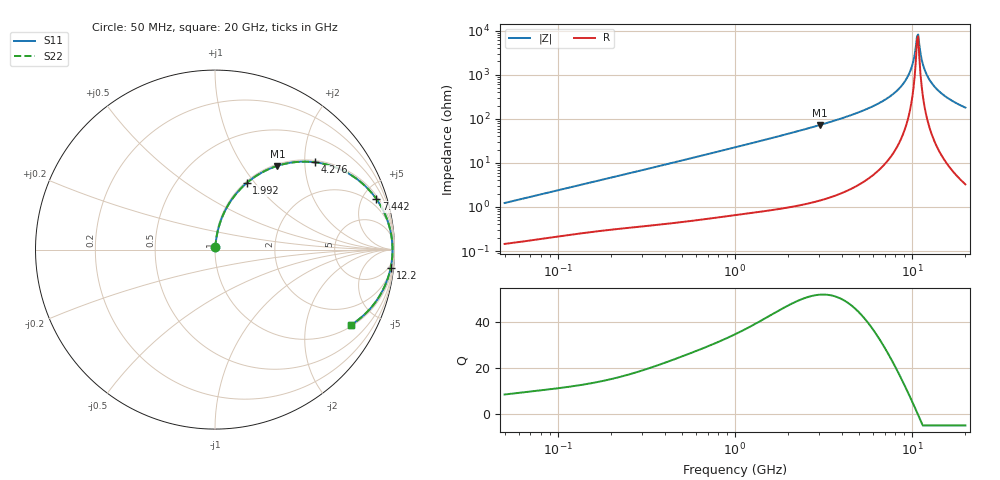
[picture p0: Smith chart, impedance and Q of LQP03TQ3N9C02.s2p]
!Murata Part Number: LQP03TQ3N9C02
!These Parameters are Measured in Series Mode Connection
!  o--[Z]--o
!Port1  Port2
!  o-------o
!Freq. Start=50[MHz] Stop=20[GHz], 401[Steps]
# Hz S RI R 50
!Freq.(Hz) S11(Real) S11(Imag) S21(Real) S21(Imag) S12(Real) S12(Imag) S22(Real) S22(Imag)
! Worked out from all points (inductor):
!   401 points, 50 MHz to 20 GHz, reference 50 ohm
!   read as one part in series: L = 3.84 nH near 51.52 MHz
!   highest Q = 51.7 at 3.03 GHz (marker M1), where L = 3.81 nH
!   self-resonance near 10.66 GHz
!   S11 on the Smith chart (normalised r, x): 50 MHz: 1.00, +0.02; 1.992 GHz: 1.02, +0.91; 4.276 GHz: 1.05, +2.24; 7.442 GHz: 1.25, +6.28; 12.2 GHz: 3, -19; 20 GHz: 1.06, -3.58
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5e7  0.00159 0.0122  0.9984 -0.0122  0.9984 -0.0122  0.00159 0.0122
1.364002e8  0.00353 0.0317  0.9965 -0.0317  0.9965 -0.0317  0.00353 0.0317
3.721004e8  0.0109 0.083  0.9891 -0.083  0.9891 -0.083  0.0109 0.083
1e9  0.0535 0.2111  0.9465 -0.2111  0.9465 -0.2111  0.0535 0.2111
1.99176e9  0.1772 0.3713  0.8228 -0.3713  0.8228 -0.3713  0.1772 0.3713
2.728004e9  0.2962 0.4469  0.7038 -0.4469  0.7038 -0.4469  0.2962 0.4469
3.029571e9  0.3477 0.4667  0.6523 -0.4667  0.6523 -0.4667  0.3477 0.4667
4.275624e9  0.5547 0.4868  0.4453 -0.4868  0.4453 -0.4868  0.5547 0.4868
5.856089e9  0.7646 0.4113  0.2354 -0.4113  0.2354 -0.4113  0.7646 0.4113
7.442007e9  0.8988 0.2824  0.1012 -0.2824  0.1012 -0.2824  0.8988 0.2824
8.516016e9  0.9514 0.1872  0.0486 -0.1872  0.0486 -0.1872  0.9514 0.1872
9.457416e9  0.9773 0.1053  0.0227 -0.1053  0.0227 -0.1053  0.9773 0.1053
1.004137e10  0.9855 0.0567  0.0145 -0.0567  0.0145 -0.0567  0.9855 0.0567
1.050288e10  0.9885 0.0197  0.0115 -0.0197  0.0115 -0.0197  0.9885 0.0197
1.066139e10  0.9889 0.00735  0.0111 -0.00735  0.0111 -0.00735  0.9889 0.00735
1.082228e10  0.989 -0.00502  0.011 0.00502  0.011 0.00502  0.989 -0.00502
1.098561e10  0.9888 -0.0174  0.0112 0.0174  0.0112 0.0174  0.9888 -0.0174
1.149051e10  0.9862 -0.0544  0.0138 0.0544  0.0138 0.0544  0.9862 -0.0544
1.220001e10  0.9784 -0.1032  0.0216 0.1032  0.0216 0.1032  0.9784 -0.1032
1.334722e10  0.9578 -0.1741  0.0422 0.1741  0.0422 0.1741  0.9578 -0.1741
1.482269e10  0.9212 -0.2512  0.0788 0.2512  0.0788 0.2512  0.9212 -0.2512
2e10  0.7584 -0.4191  0.2416 0.4191  0.2416 0.4191  0.7584 -0.4191
